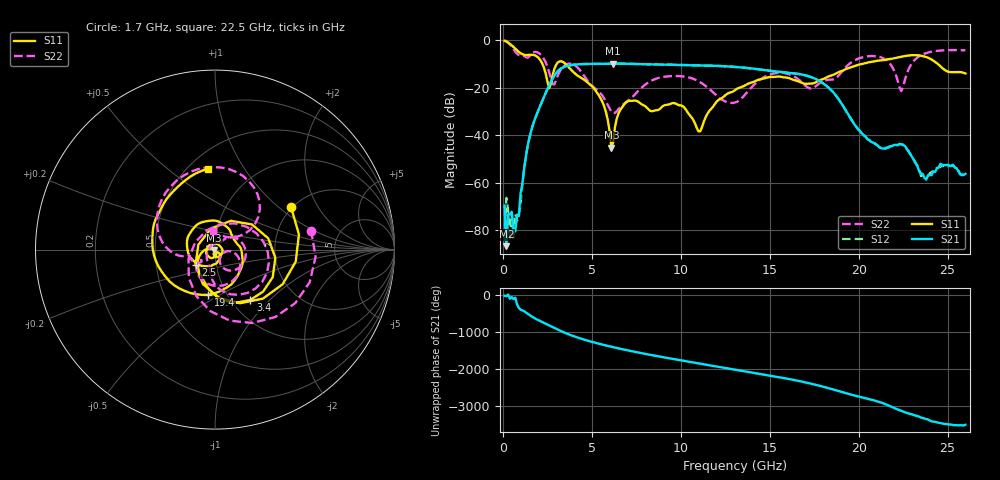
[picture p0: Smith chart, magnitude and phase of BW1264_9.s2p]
!Keysight Technologies,N5245B,MY57181159,A.13.60.06
!Date: Friday, December 18, 2020 23:52:24
!Correction: S11(Full 2 Port(1,2))
!S21(Full 2 Port(1,2))
!S12(Full 2 Port(1,2))
!S22(Full 2 Port(1,2))
!S2P File: Measurements: S11, S21, S12, S22:
# Hz S  dB  R 50
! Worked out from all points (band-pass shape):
!   260 points, 100 MHz to 26 GHz, reference 50 ohm
!   highest |S21| = -9.95 dB at 6.2 GHz (marker M1); lowest = -86.6 dB at 200 MHz (marker M2)
!   |S21| within 3 dB of the highest: 3.11 GHz to 15.01 GHz (11.9 GHz wide, 131 % of centre)
!   lowest |S11| = -45.2 dB at 6.1 GHz (marker M3), VSWR 1.01, Z = 49.5 - j0.168 ohm
!   |S11| at or under -10 dB: 2.221 GHz to 3.037 GHz (816 MHz wide, 31 % of centre); 3.515 GHz to 20.23 GHz (16.72 GHz wide, 141 % of centre); 24.44 GHz to end of sweep
!   |S22| runs from -30.7 to -0.2 dB; largest |S21 - S12| = 0.00053
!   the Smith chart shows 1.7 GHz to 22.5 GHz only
!   S11 on the Smith chart (normalised r, x): 1.7 GHz: 1.96, +1.22; 2.5 GHz: 0.79, -0.14; 3.4 GHz: 1.22, -0.77; 19.4 GHz: 0.82, -0.44; 22.5 GHz: 0.62, +0.70
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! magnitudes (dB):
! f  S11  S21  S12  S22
! 100 MHz  -0.4  -69.6  -84.6  -0.2
! 200 MHz  -0.7  -86.6  -66.3  -0.6
! 400 MHz  -1.6  -73.3  -84.3  -1.9
! 800 MHz  -4.3  -73.4  -76.1  -5.8
! 1.7 GHz  -6.3  -35.5  -35.5  -5.3
! 2.5 GHz  -17.2  -20.7  -20.8  -11.1
! 3.4 GHz  -9.3  -11.5  -11.5  -11.2
! 4.5 GHz  -16.3  -10.1  -10.1  -14.4
! 5.6 GHz  -26.1  -10.0  -10.0  -23.4
! 6.1 GHz  -45.2  -10.0  -10.0  -30.2
! 6.2 GHz  -43.0  -9.9  -10.0  -30.7
! 7 GHz  -25.9  -10.0  -10.0  -25.7
! 8.8 GHz  -29.1  -10.3  -10.3  -15.9
! 11.1 GHz  -38.4  -10.7  -10.7  -17.8
! 13.1 GHz  -20.8  -11.3  -11.3  -26.1
! 15.3 GHz  -15.5  -13.2  -13.2  -14.0
! 17.4 GHz  -18.3  -15.8  -15.8  -20.3
! 19.4 GHz  -11.9  -31.1  -31.1  -10.5
! 21.7 GHz  -8.1  -44.8  -45.2  -9.4
! 22.5 GHz  -6.9  -44.0  -44.3  -19.6
! 23.8 GHz  -7.2  -58.7  -56.8  -5.5
! 26 GHz  -14.1  -56.2  -56.6  -4.3
